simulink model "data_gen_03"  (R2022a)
settings: Solver=VariableStepAuto  StartTime=0.0  StopTime=300  RelTol=1e-3
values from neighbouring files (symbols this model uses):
  C = 6.3000e-04    (= 0.00063)    [maglev_init.m]
  g = 9.80    (= 9.8)    [maglev_init.m]
  K = 1.0e+03 * [-2.4567   -0.1235    0.0237]    [maglev_init.m]
  L1 = 0.6000    (= 0.6)    [maglev_init.m]
  m = 0.0300    (= 0.03)    [maglev_init.m]
  mpert = 0    [maglev_init.m]
  R = 45    [maglev_init.m]
  Ts = 0.005    [maglev_init.m]    (also in train_net.m)
  x1_0 = 0.1    [maglev_init.m]
  x1_d = 0.05    [maglev_init.m]
  x2_0 = 0    [maglev_init.m]
  x2_d = 0    [maglev_init.m]
  x3_0 = 0.2    [maglev_init.m]

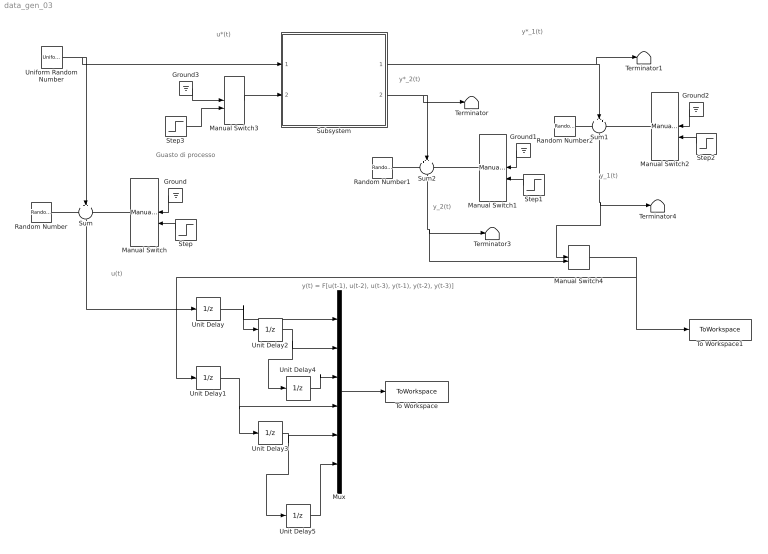
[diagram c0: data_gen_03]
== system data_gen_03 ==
  note: y(t) = F[u(t-1), u(t-2), u(t-3), y(t-1), y(t-2), y(t-3)]
  note: y_2(t)
  note: y*_1(t)
  note: u(t)
  note: y*_2(t)
  note: y_1(t)
  note: u*(t)
  note: Guasto di processo
  Ground{,1..3} (4 alike) : Ground
  Manual Switch{,1..3} (4 alike) : ManualSwitch
  Manual Switch4 : ManualSwitch  CurrentSetting=0
  Mux : Mux  Inputs=6
  Random Number : RandomNumber  Variance=1e-9  Seed=1  SampleTime=Ts
  Random Number1 : RandomNumber  Variance=1e-6  Seed=3  SampleTime=Ts
  Random Number2 : RandomNumber  Variance=1e-9  Seed=2  SampleTime=Ts
  Step : Step  Time=150  SampleTime=0
  Step1 : Step  Time=150  SampleTime=0
  Step2 : Step  Time=150  SampleTime=0
  Step3 : Step  Time=15  After=2*R  SampleTime=0
  Subsystem : Subsystem
  Sum : Sum  Inputs=+++
  Sum1 : Sum  Inputs=+++
  Sum2 : Sum  Inputs=+++
  Terminator{,1,3..4} (4 alike) : Terminator
  To Workspace : ToWorkspace  VariableName=Psim  SampleTime=Ts
  To Workspace1 : ToWorkspace  VariableName=Tsim  SampleTime=Ts
  Uniform Random Number : UniformRandomNumber  Minimum=x1_d*0.9  Maximum=x1_d*1.1  Seed=1  SampleTime=0.5
  Unit Delay{,1..5} (6 alike) : UnitDelay  SampleTime=Ts  HasFrameUpgradeWarning=on
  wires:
  Subsystem/1(Out1) -> Terminator1/1, Sum1/2
  Subsystem/2(Out2) -> Terminator/1, Sum2/2
  Random Number/1 -> Sum/1
  Manual Switch/1 -> Sum/3
  Manual Switch2/1 -> Sum1/3
  Manual Switch1/1 -> Sum2/3
  Random Number1/1 -> Sum2/1
  Ground/1 -> Manual Switch/1
  Step/1 -> Manual Switch/2
  Ground1/1 -> Manual Switch1/1
  Step1/1 -> Manual Switch1/2
  Sum2/1 -> Manual Switch4/2, Terminator3/1
  Random Number2/1 -> Sum1/1
  Ground2/1 -> Manual Switch2/1
  Step2/1 -> Manual Switch2/2
  Manual Switch3/1 -> Subsystem/2(fs)
  Ground3/1 -> Manual Switch3/1
  Uniform Random Number/1 -> Subsystem/1(u), Sum/2
  Step3/1 -> Manual Switch3/2
  Sum/1 -> Unit Delay/1
  Unit Delay/1 -> Unit Delay2/1, Mux/1
  Unit Delay1/1 -> Mux/4, Unit Delay3/1
  Mux/1 -> To Workspace/1
  Sum1/1 -> Manual Switch4/1, Terminator4/1
  Manual Switch4/1 -> To Workspace1/1, Unit Delay1/1
  Unit Delay2/1 -> Unit Delay4/1, Mux/2
  Unit Delay3/1 -> Unit Delay5/1, Mux/5
  Unit Delay4/1 -> Mux/3
  Unit Delay5/1 -> Mux/6

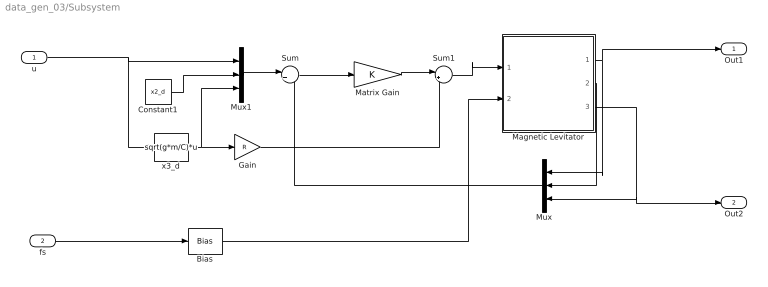
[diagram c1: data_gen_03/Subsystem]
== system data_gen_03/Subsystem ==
  u : Inport
  fs : Inport  Port=2
  Bias : Bias  Bias=R
  Constant1 : Constant  Value=x2_d
  Gain : Gain  Gain=R
  Magnetic Levitator : Subsystem  mask{m=m+mpert, R=R, L1=L1, C=C, g=g}
      mask prompts: m "ball's mass (m)"; R "Electromagnet's resistance (R)"; L1 "Electromagnet's inductance (L1)"; C "Magnetic force constant (C)"; g "Gravitational acceleration (g)"
  Matrix Gain : Gain  Gain=K  Multiplication=Matrix(K*u)  SaturateOnIntegerOverflow=on
  Mux : Mux  Inputs=3
  Mux1 : Mux  Inputs=3
  Sum : Sum  Inputs=|+-  InputSameDT=on  SaturateOnIntegerOverflow=on
  Sum1 : Sum  Inputs=|++  InputSameDT=on  SaturateOnIntegerOverflow=on
  x3_d : Fcn  Expr=sqrt(g*m/C)*u
  Out1 : Outport
  Out2 : Outport  Port=2
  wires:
  u/1 -> x3_d/1, Mux1/1
  Magnetic Levitator/2(x2) -> Mux/2
  x3_d/1 -> Mux1/3, Gain/1
  Mux1/1 -> Sum/1
  Gain/1 -> Sum1/2
  Mux/1 -> Sum/2
  Constant1/1 -> Mux1/2
  Sum/1 -> Matrix Gain/1
  Sum1/1 -> Magnetic Levitator/1(u)
  Magnetic Levitator/1(x1) -> Out1/1, Mux/1
  Magnetic Levitator/3(x3) -> Out2/1, Mux/3
  Matrix Gain/1 -> Sum1/1
  Bias/1 -> Magnetic Levitator/2(fs)
  fs/1 -> Bias/1

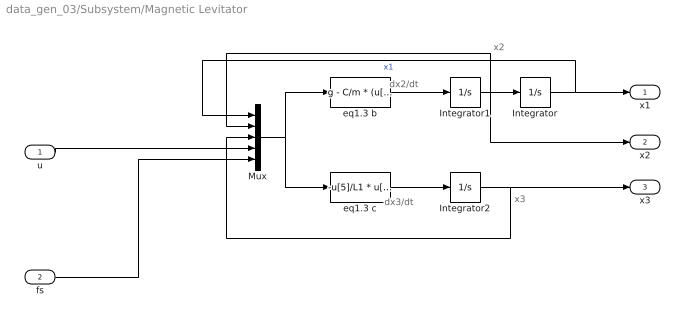
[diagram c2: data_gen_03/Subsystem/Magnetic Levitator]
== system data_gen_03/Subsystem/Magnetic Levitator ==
  note: x2
  note: x3
  note: dx2/dt
  note: dx3/dt
  u : Inport
  fs : Inport  Port=2
  Integrator : Integrator  InitialCondition=x1_0
  Integrator1 : Integrator  InitialCondition=x2_0
  Integrator2 : Integrator  InitialCondition=x3_0
  Mux : Mux  Inputs=5
  eq1.3 b : Fcn  Expr=g - C/m * (u[3] / u[1])^2
  eq1.3 c : Fcn  Expr=-u[5]/L1 * u[3] + (2*C)/L1 * ( u[2] * u[3] / u[1]^2 ) + 1/L1 * u[4]
  x1 : Outport
  x2 : Outport  Port=2
  x3 : Outport  Port=3
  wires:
  eq1.3 b/1 -> Integrator1/1
  Integrator1/1 -> Integrator/1, Mux/2, x2/1
  eq1.3 c/1 -> Integrator2/1
  Mux/1 -> eq1.3 b/1, eq1.3 c/1
  Integrator/1 -> Mux/1, x1/1  "x1"
  Integrator2/1 -> Mux/3, x3/1
  u/1 -> Mux/4
  fs/1 -> Mux/5
